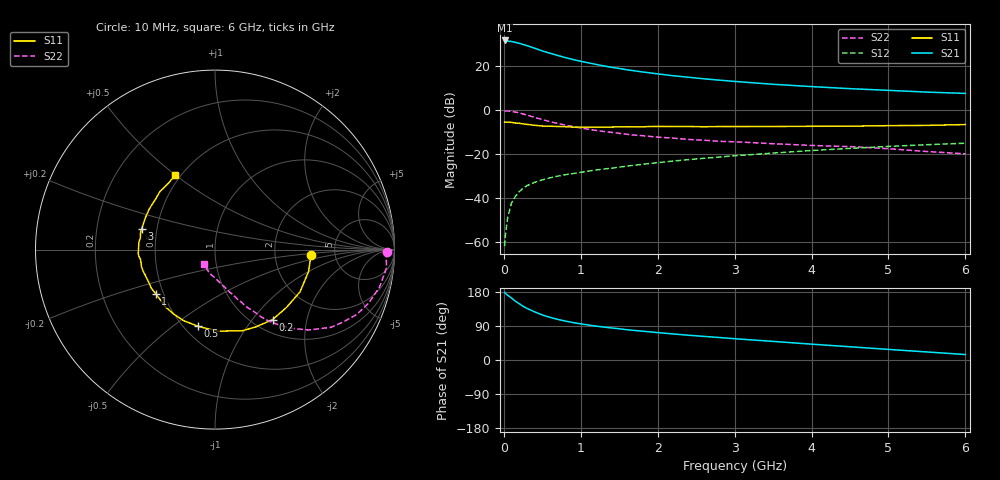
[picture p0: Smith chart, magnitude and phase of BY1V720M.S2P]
! SIEMENS Small Signal Semiconductors
! BFY420
! Si NPN RF SIEGET Grounded Emitter Transistor in MICRO-X
! VCE = 1.75 V  IC = 20 mA
! Common Emitter S-Parameters:  October  1996
# GHz  S  MA  R  50
!  f  S11  S21  S12  S22
! GHz  MAG  ANG  MAG  ANG  MAG  ANG  MAG  ANG
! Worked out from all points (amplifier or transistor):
!   36 points, 10 MHz to 6 GHz, reference 50 ohm
!   highest |S21| = 31.8 dB at 10 MHz (marker M1)
!   |S21| within 3 dB of that: start of sweep to 353.3 MHz
!   unconditionally stable (mu >= 1): 1.953 GHz to end of sweep
!   at 250 MHz: K = 0.30, MSG = 32.8 dB, |S12| = -35.6 dB
!   at 1.4 GHz: K = 0.92, MSG = 23.0 dB, |S12| = -26.4 dB
!   at 6 GHz: K = 1.08, MAG = 9.6 dB, |S12| = -15.0 dB
!   S11 on the Smith chart (normalised r, x): 10 MHz: 3.29, -0.27; 200 MHz: 1.22, -1.27; 500 MHz: 0.59, -0.62; 1 GHz: 0.45, -0.27; 3 GHz: 0.41, +0.12; 6 GHz: 0.47, +0.50
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0.01  0.5369 -3.1  38.91 178.8  0.0008 115.1  0.9576 -0.7
0.02  0.534 -5.6  38.58 175.8  0.0014 93.2  0.9551 -2.0
0.05  0.5355 -13.2  37.62 171.0  0.0036 82.2  0.9607 -6.2
0.1  0.5289 -26.5  36.84 163.5  0.0077 82.7  0.9399 -12.9
0.15  0.5123 -38.9  35.15 155.0  0.0109 74.6  0.907 -19.1
0.2  0.505 -50.5  33.55 148.6  0.014 72.4  0.8695 -24.5
0.25  0.4875 -61.8  31.57 141.8  0.0166 67.2  0.8206 -29.4
0.3  0.477 -71.6  29.6 136.2  0.0191 64.8  0.7782 -33.8
0.4  0.4543 -88.4  25.86 127.1  0.0228 61.6  0.6884 -40.6
0.5  0.4377 -102.4  22.47 118.8  0.0259 58.5  0.6125 -45.7
0.6  0.4328 -113.6  19.9 112.6  0.0289 57.0  0.5514 -49.6
0.7  0.4265 -122.5  17.74 107.2  0.0315 57.3  0.5007 -52.9
0.8  0.4222 -131.2  15.82 102.7  0.034 55.2  0.4578 -55.4
1  0.4122 -143.3  13.04 95.4  0.0385 56.1  0.3944 -58.8
1.1  0.4149 -148.9  12.02 92.3  0.041 56.6  0.3694 -60.8
1.6  0.4204 -166.9  8.361 79.9  0.0535 55.9  0.2831 -67.2
2.2  0.4258 178.9  6.118 68.8  0.0696 54.6  0.2314 -73.5
3  0.4247 164.3  4.535 56.2  0.0917 50.5  0.1913 -80.5
3.5  0.4265 155.6  3.905 49.1  0.1057 47.3  0.1728 -85.2
4.5  0.4335 140.5  3.102 34.9  0.1351 38.9  0.1484 -94.8
5.5  0.4517 125.0  2.591 21.2  0.164 29.6  0.1148 -113.5
6  0.4719 117.8  2.419 14.4  0.1775 24.7  0.1018 -127.8
